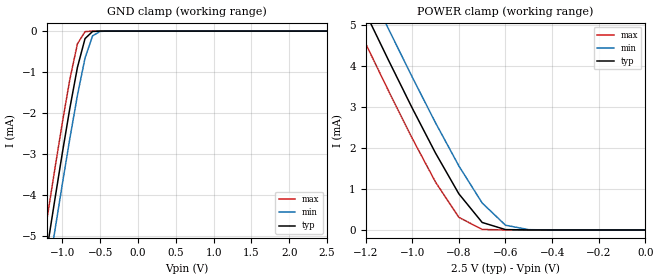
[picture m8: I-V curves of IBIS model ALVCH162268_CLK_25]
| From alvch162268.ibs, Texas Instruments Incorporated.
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|************* ALVCH162268 INPUT (2.5 V) MODEL**************
[Model]   ALVCH162268_CLK_25
Model_type  Input
Polarity   Non-Inverting
Vinl = 0.7V
Vinh = 1.7V
| variable   typ   min   max
C_comp   2.15pF   NA   NA
[Temperature Range]   50   100   0
[Voltage range]   2.5   2.3   2.7
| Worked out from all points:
|   GND clamp passes 1 mA (typ) near -0.81 V on its own axis
|   POWER clamp passes 1 mA (typ) near -0.81 V on its own axis
|Process range|   weak   strong
[GND Clamp]
|   50C:2.5V:   100C:2.3V:weak   0C:2.7V:strong
|   Voltage   I(typ)   I(min)   I(max)
-2.5V     -21.29mA   -22.02mA   -20.58mA
-1.3V     -6.503mA   -7.266mA   -5.756mA
-1.2V     -5.308mA   -6.072mA   -4.559mA
-1.1V     -4.131mA   -4.895mA   -3.383mA
-1V       -2.981mA   -3.739mA   -2.24mA
-900mV    -1.879mA   -2.62mA    -1.171mA
-800mV    -884.1uA   -1.566mA   -309.4uA
-700mV    -183.9uA   -659.5uA   -12.88uA
-600mV    -8.941uA   -116.2uA   -211.8nA
-500mV    -274.5nA   -7.235uA   -3.35nA
2.5V      4.745pA    817.5pA    4.299pA
[POWER Clamp]
|   50C:2.5V:   100C:2.3V:weak   0C:2.7V:strong
|   Voltage   I(typ)   I(min)   I(max)
-2.5V     21.29mA    22.02mA    20.58mA
-1.3V     6.503mA    7.266mA    5.756mA
-1.2V     5.308mA    6.072mA    4.559mA
-1.1V     4.131mA    4.895mA    3.382mA
-1V       2.98mA     3.739mA    2.24mA
-900mV    1.879mA    2.62mA     1.171mA
-800mV    884.1uA    1.566mA    309.4uA
-700mV    183.9uA    659.4uA    12.88uA
-600mV    8.941uA    116.1uA    211.8nA
-500mV    274.5nA    7.235uA    3.35nA
0V        4.745pA    6.413pA    4.996pA
